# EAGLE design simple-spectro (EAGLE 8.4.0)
DELETE: MF
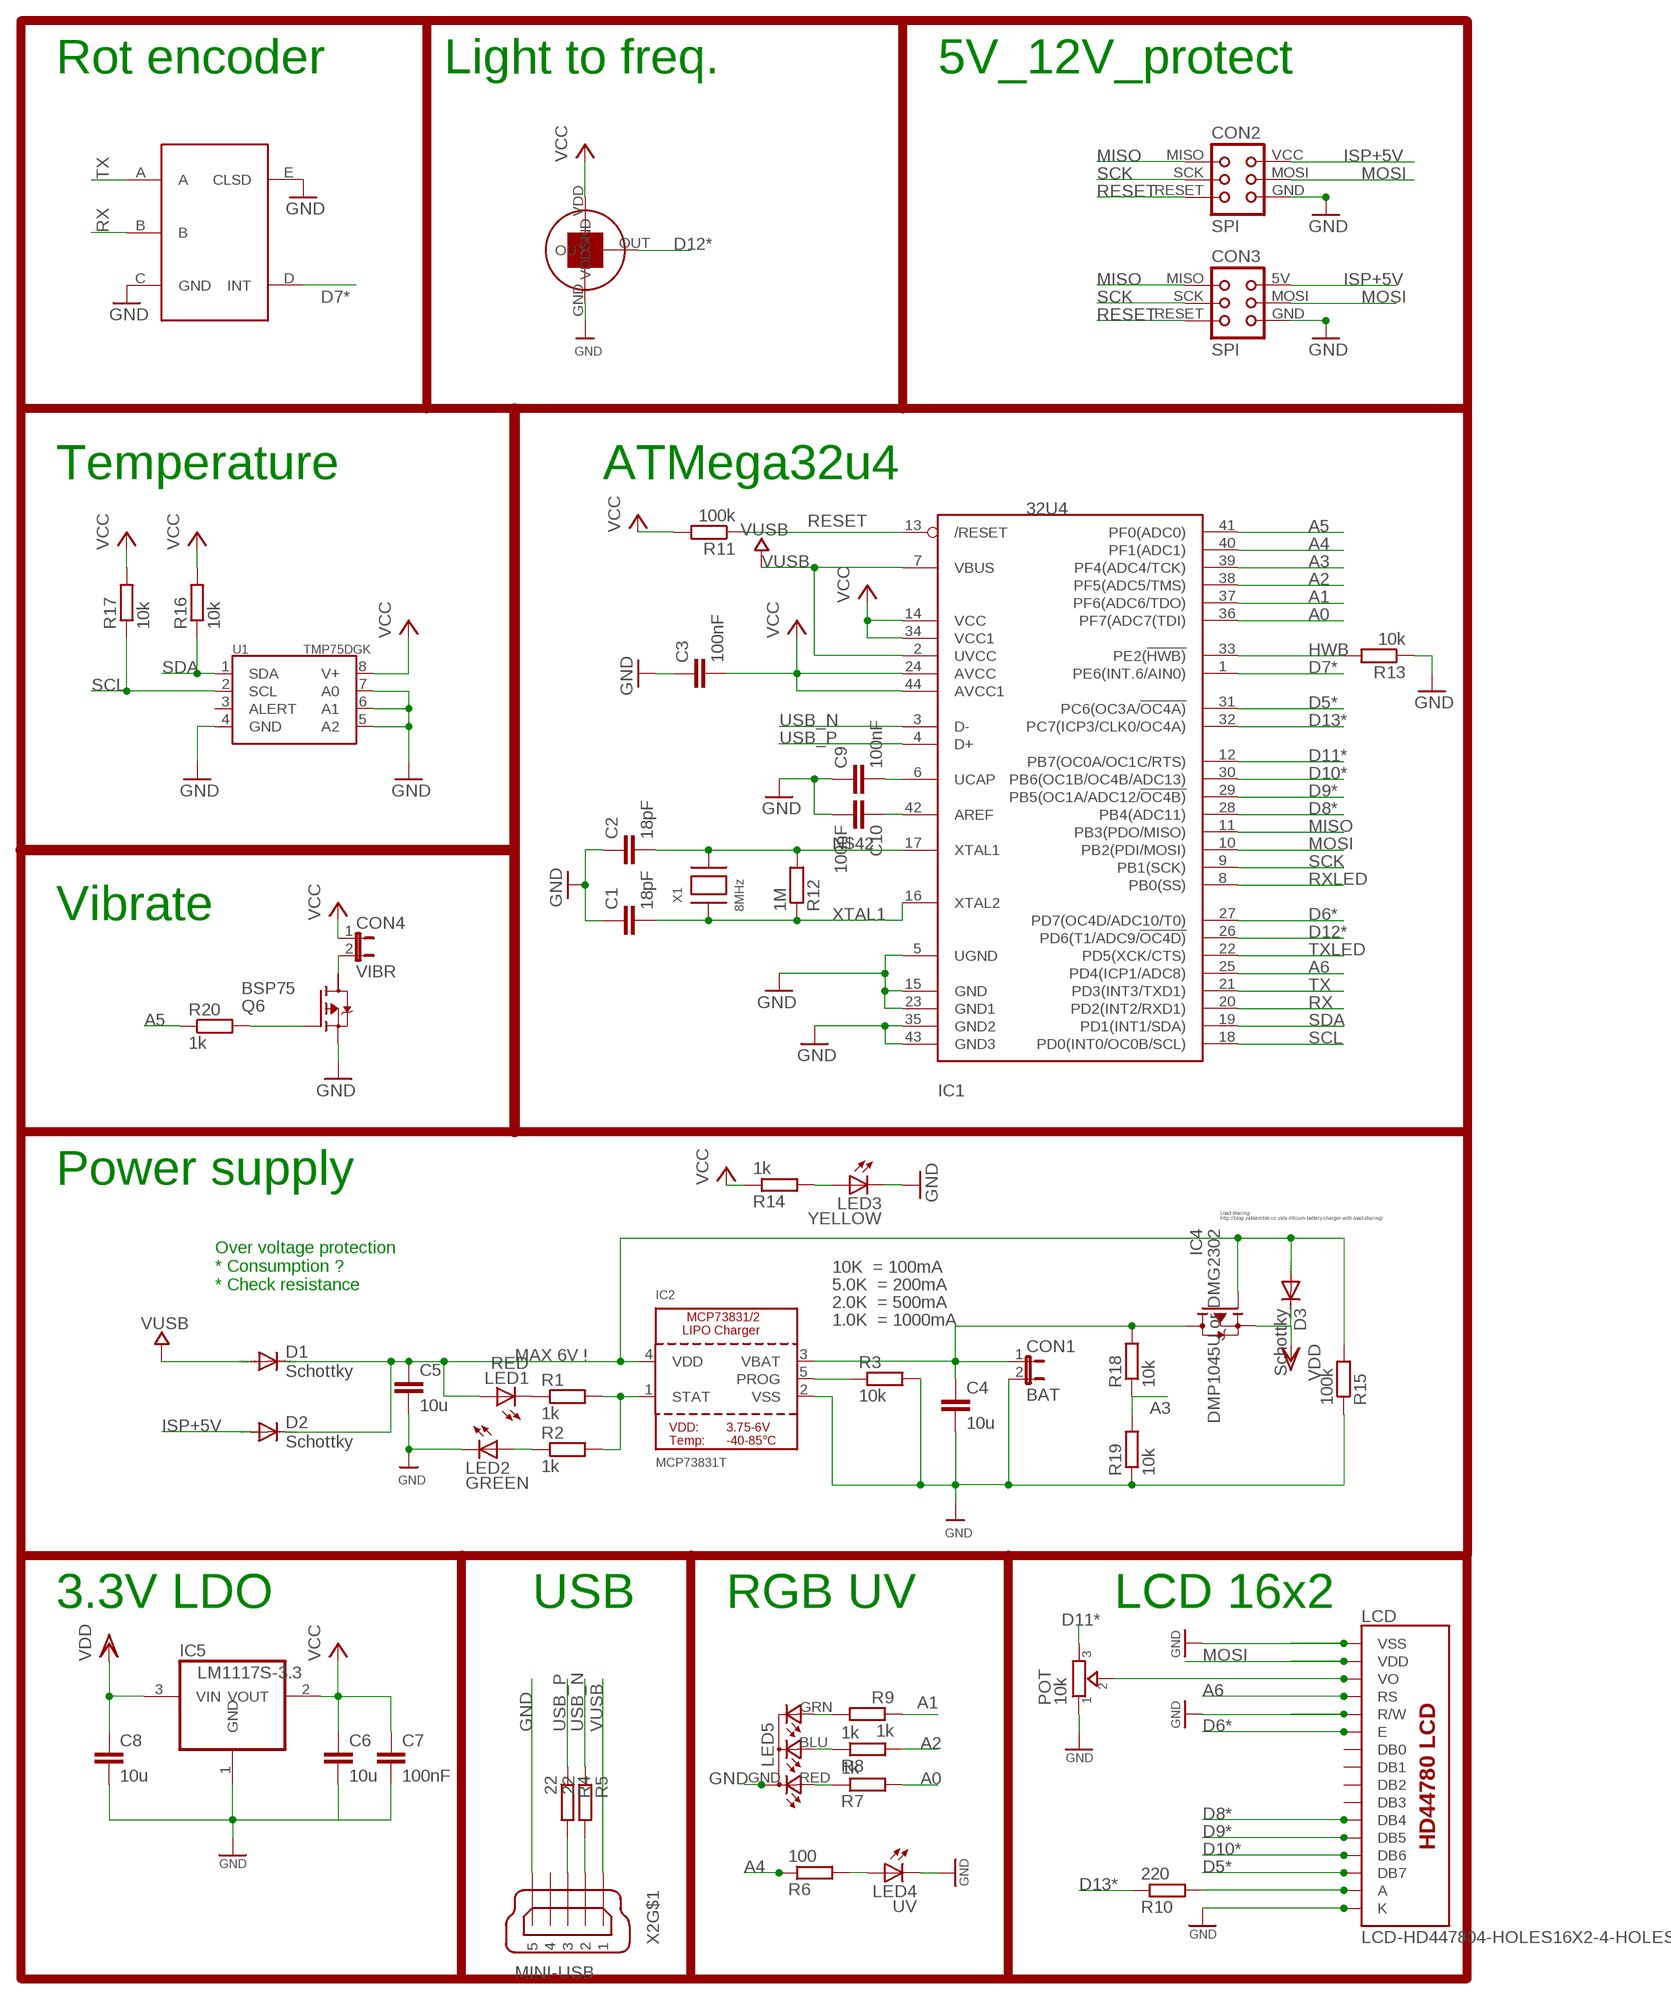
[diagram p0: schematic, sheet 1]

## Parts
C1  18pF  C-EUC0805K  [C0805K]
C2  18pF  C-EUC0805K  [C0805K]
C3  100nF  C-EUC0805K  [C0805K]
C4  10u  C-EUC0805K  [C0805K]
C5  10u  C-EUC0805K  [C0805K]
C6  10u  C-EUC0805K  [C0805K]
C7  100nF  C-EUC0805K  [C0805K]
C8  10u  C-EUC0805K  [C0805K]
C9  100nF  C-EUC0805K  [C0805K]
C10  100nF  C-EUC0805K  [C0805K]
CON1  BAT  JP1E  [JP1]
CON2  SPI  TINYISP  [TINYISP]
CON3  SPI  TINYISPT  [TC2030-MCP-NL]
CON4  VIBR  JP1E  [JP1]
D1  Schottky  MBR0520LT  [SOD123]
D2  Schottky  MBR0520LT  [SOD123]
D3  Schottky  MBR0520LT  [SOD123]
IC1  32U4  ATMEGA32U4-AU  [TQFP44]
IC2  MCP73831T  MCP73831/2  [SOT23-5]
IC4  DMP1045U or DMG2302  TRANSISTOR_FET_TSM2301CX  [SOT-23]
IC5  LM1117S-3.3  REG1117  [SOT223]
LCD  LCD-HD447804-HOLES16X2-4-HOLES  [LCD-16X2-4HOLES]
LED1  RED  LED1206  [LED-1206]
LED2  GREEN  LED1206  [LED-1206]
LED3  YELLOW  LED1206  [LED-1206]
LED4  UV  LED5MM  [LED5MM]
LED5  RGB-COMMON-CATHODE  [LED-TRICOLOR-THROUGHHOLE]
POT  10k  TRIMMER-3362P  [TRIMMER_3362P]
Q6  BSP75  BSP613P  [PG-SOT-223]
R1  1k  R-EU_R0805  [R0805]
R2  1k  R-EU_R0805  [R0805]
R3  10k  R-EU_R0805  [R0805]
R4  22  R-EU_R0805  [R0805]
R5  22  R-EU_R0805  [R0805]
R6  100  R-EU_R0805  [R0805]
R7  1k  R-EU_R0805  [R0805]
R8  1k  R-EU_R0805  [R0805]
R9  1k  R-EU_R0805  [R0805]
R10  220  R-EU_R0805  [R0805]
R11  100k  R-EU_R0805  [R0805]
R12  1M  R-EU_R0805  [R0805]
R13  10k  R-EU_R0805  [R0805]
R14  1k  R-EU_R0805  [R0805]
R15  100k  R-EU_R0805  [R0805]
R16  10k  R-EU_R0805  [R0805]
R17  10k  R-EU_R0805  [R0805]
R18  10k  R-EU_R0805  [R0805]
R19  10k  R-EU_R0805  [R0805]
R20  1k  R-EU_R0805  [R0805]
U1  TMP75DGK  [MSOP8]
U$1  EC11E  [EC11E]
U$7  TSL237  [TSL237]
X1  8MHz  XTALNX6035  [NX6035]
X2  MINI-USB  MINI-USB-SCHIELD-32005-201  [32005-201]

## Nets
A0: IC1.36(PF7(ADC7(TDI)) R7.2
A1: IC1.37(PF6(ADC6/TDO)) R9.1
A2: IC1.38(PF5(ADC5/TMS)) R8.2
A3: IC1.39(PF4(ADC4/TCK)) R18.1 R19.2
A4: IC1.40(PF1(ADC1)) R6.1
A5: IC1.41(PF0(ADC0)) R20.1
A6: IC1.25(PD4(ICP1/ADC8)) LCD.4(RS)
AREF: C10.1 IC1.42(AREF)
D5*: IC1.31(PC6(OC3A/!OC4A)) LCD.14(DB7)
D6*: IC1.27(PD7(OC4D/ADC10/T0)) LCD.6(E)
D7*: IC1.1(PE6(INT.6/AIN0)) U$1.D(INT)
D8*: IC1.28(PB4(ADC11)) LCD.11(DB4)
D9*: IC1.29(PB5(OC1A/ADC12/!OC4B)) LCD.12(DB5)
D10*: IC1.30(PB6(OC1B/OC4B/ADC13)) LCD.13(DB6)
D11*: IC1.12(PB7(OC0A/OC1C/RTS)) POT.3
D12*: IC1.26(PD6(T1/ADC9/!OC4D)) U$7.OUT
D13*: IC1.32(PC7(ICP3/CLK0/OC4A)) R10.1
GND [power]: C1.1 C2.1 C3.1 C4.2 C5.2 C6.2 C7.2 C8.2 C9.1 C10.2 CON1.2 CON2.GND CON3.GND IC1.5(UGND) IC1.15(GND) IC1.23(GND1) IC1.35(GND2) IC1.43(GND3) IC2.2(VSS) IC5.1(GND) LCD.1(VSS) LCD.5(R/W) LCD.16(K) LED2.C LED3.C LED4.K(C) LED5.GND(A2) POT.1 Q6.3(S) R3.2 R13.1 R15.1 R19.1 U1.4(GND) U1.5(A2) U1.6(A1) U1.7(A0) U$1.C(GND) U$1.E(CLSD) U$7.GND X2.5
HWB: IC1.33(PE2(!HWB)) R13.2
ISP+5V: CON2.VCC CON3.5V(VCC) D2.A
MISO: CON2.MISO CON3.MISO IC1.11(PB3(PDO/MISO))
MOSI: CON2.MOSI CON3.MOSI IC1.10(PB2(PDI/MOSI)) LCD.2(VDD)
N$1: C9.2 IC1.6(UCAP)
N$2: LCD.3(VO) POT.2
N$3: LED4.A R6.2
N$4: LED1.C R1.1
N$5: IC2.1(STAT) R1.2 R2.2
N$6: IC2.5(PROG) R3.1
N$7: LED2.A R2.1
N$8: Q6.1(G) R20.2
N$9: LED5.GRN(CGREEN) R9.2
N$10: LED5.BLU(CBLUE) R8.1
N$11: LCD.15(A) R10.2
N$12: LED3.A R14.2
N$13: LED5.RED(CRED) R7.1
N$14: CON4.2 Q6.2(D)
N$15: C5.1 D1.C D2.C D3.A IC2.4(VDD) IC4.1(G) LED1.A R15.2
N$42: C2.2 IC1.17(XTAL1) R12.2 X1.P$2
RESET: CON2.RESET CON3.RESET IC1.13(/RESET) R11.1
RX: IC1.20(PD2(INT2/RXD1)) U$1.B
RXLED: IC1.8(PB0(SS))
SCK: CON2.SCK CON3.SCK IC1.9(PB1(SCK))
SCL: IC1.18(PD0(INT0/OC0B/SCL)) R17.1 U1.2(SCL)
SDA: IC1.19(PD1(INT1/SDA)) R16.1 U1.1(SDA)
TX: IC1.21(PD3(INT3/TXD1)) U$1.A
TXLED: IC1.22(PD5(XCK/CTS))
USB_N: IC1.3(D-) R5.1
USB_P: IC1.4(D+) R4.1
USBC_N: R5.2 X2.2
USBC_P: R4.2 X2.3
VBAT1: C4.1 CON1.1 IC2.3(VBAT) IC4.3(D) R18.2
VCC: C3.2 C6.1 C7.1 CON4.1 IC1.14(VCC) IC1.24(AVCC) IC1.34(VCC1) IC1.44(AVCC1) IC5.2(VOUT) R11.2 R14.1 R16.2 R17.2 U1.8(V+) U$7.VDD
VDD [power]: C8.1 D3.C IC4.2(S) IC5.3(VIN)
VUSB: D1.A IC1.2(UVCC) IC1.7(VBUS) X2.1
XTAL1: C1.2 IC1.16(XTAL2) R12.1 X1.P$1
Unconnected: LCD.7(DB0) LCD.8(DB1) LCD.9(DB2) LCD.10(DB3) Q6.4(D) U1.3(ALERT) X2.4 X2.M1(S:S1) X2.M2(S:S2) X2.M3(S:S3) X2.M4(S:S4)

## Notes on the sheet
- Rot encoder | Light to freq. | 5V_12V_protect
- Temperature | ATMega32u4
- Vibrate
- Power supply
- Load sharing:
  http://blog.zakkemble.co.uk/a-lithium-battery-charger-with-load-sharing/
- 10K  = 100mA
- Over voltage protection
  * Consumption ?
  * Check resistance
- 5.0K  = 200mA
- 2.0K  = 500mA
- 1.0K  = 1000mA
- MAX 6V !
- 3.3V LDO | USB | RGB UV | LCD 16x2

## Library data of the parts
C1 C2 = rcl:C-EU: CAPACITOR, European symbol; ELECROW: C1797; LCSC: C1797; MPN: 77-VJ1206A180JXXPBC
C3 C9 C10 = rcl:C-EU: CAPACITOR, European symbol; ELECROW: C49678; LCSC: C49678; MPN: 80-C1206C104K5R
C4-C6 C8 = rcl:C-EU: CAPACITOR, European symbol; ELECROW: C15850; LCSC: C15850; MPN: 77-VJ1206V106ZXQTBC
C7 = rcl:C-EU: CAPACITOR, European symbol; ELECROW: C49678; LCSC: C77502; MPN: 80-C1206C104K5R
CON1 CON4 = jumper:JP1E: JUMPER
CON2 = lpatiny:TINYISP: CONNECTOR; OC_FARNELL: unknown; OC_NEWARK: unknown
CON3 = lpatiny:TINYISP: CONNECTOR
D1-D3 = diode:MBR0520LT: SCHOTTKY BARRIER RECTIFIER; LCSC: C82544; MPN: 621-1N5819HW-F
IC1 = adafruit:ATMEGA32U4: http://www.ladyada.net/library/eagle; LCSC: C44854; MPN: 556-ATMEGA32U4RC-AU
IC2 = microbuilder:MCP73831/2: MCP73831/2 LIPO Charger VDD: 3.75 - 6V Temp -40 - 85°C Programmable Charge Rate: 15-500mA NOTE: STAT is a tri-state logic output on the MCP73831 and an open-drain output on the MCP73832. SOT23-5 with 4.2V output and tri-state logic on STAT = MCP73831T-2ACI/OT; LCSC: C14879; MPN: 579-MCP73831T-3ACIOT
IC4 = dp_devices:TRANSISTOR_FET_TSM2301CX: 20V P-Channel Enhancement Mode MOSFET; LCSC: C96613; MPN: 621-DMP1045U-7
IC5 = burr-brown:REG1117: 800mA and 1A Low Dropout (LDO) Positive Regulator 1.8V, 2.5V, 2.85V, 3.3V, 5V, and Adj; LCSC: C126027; MPN: REG1117; OC_FARNELL: 1097566; OC_NEWARK: 14P6981
LCD = HD44780LCD:LCD-HD44780
LED1 = SparkFun:LED: LEDs; LCSC: C49018; MPN: 604-APT3216EC
LED2 = SparkFun:LED: LEDs; LCSC: C14641; MPN: 604-APTR3216SGC
LED3 = SparkFun:LED: LEDs; LCSC: C84273; MPN: 604-APTR3216YC
LED4 = SparkFun:LED: LEDs
LED5 = lpatiny:RGB-COMMON-CATHODE
POT = dp_devices:TRIMMER: Trimmer resistor
Q6 = infineon:BSP613P: SIPMOS (R) Small-Signal-Transistor P-Channel (2 Drain) Source: http://www.infineon.com/dgdl/BSP613P_Rev2.4.pdf; LCSC: C111029; OC_FARNELL: unknown; OC_NEWARK: unknown
R1 R2 R7-R9 R14 R20 = rcl:R-EU_: RESISTOR, European symbol; ELECROW: C17513; LCSC: C17513
R3 R13 R16-R19 = rcl:R-EU_: RESISTOR, European symbol; ELECROW: C17414; LCSC: C17414
R4 R5 = rcl:R-EU_: RESISTOR, European symbol; ELECROW: C17561; LCSC: C17561
R6 = rcl:R-EU_: RESISTOR, European symbol; ELECROW: C17408; LCSC: C17408; MPN: 667-ERJ-8GEYJ101V
R10 = rcl:R-EU_: RESISTOR, European symbol; ELECROW: C17557; LCSC: C17557
R11 R15 = rcl:R-EU_: RESISTOR, European symbol; ELECROW: C118844; LCSC: C118844; MPN: RC1206FR-07100KL
R12 = rcl:R-EU_: RESISTOR, European symbol; ELECROW: C17514; LCSC: C17514
U1 = ti_tmp:TMP75; LCSC: C94387
U$1 = lpatiny:EC11E: ALPS Rotary encoder
U$7 = lpatiny:TSL237
X1 = lpatiny:XTAL: Low cost SMT crystals, no capacitors included; LCSC: C122522; MPN: 729-F60800010
X2 = con-cypressindustries:MINI-USB-SCHIELD-: MINI USB-B Conector Source: www.cypressindustries.com; LCSC: C46391; MPN: 649-10033526-N3212LF

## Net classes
0 default: width 0.406 mm, clearance 0.25 mm
1 power: width 0.406 mm, drill 0.305 mm, clearance 0.25 mm
2 VIN: width 0.406 mm, clearance 0.25 mm
3 fine: width 0.406 mm, clearance 0.25 mm
4 aref: width 0.406 mm, clearance 0.25 mm

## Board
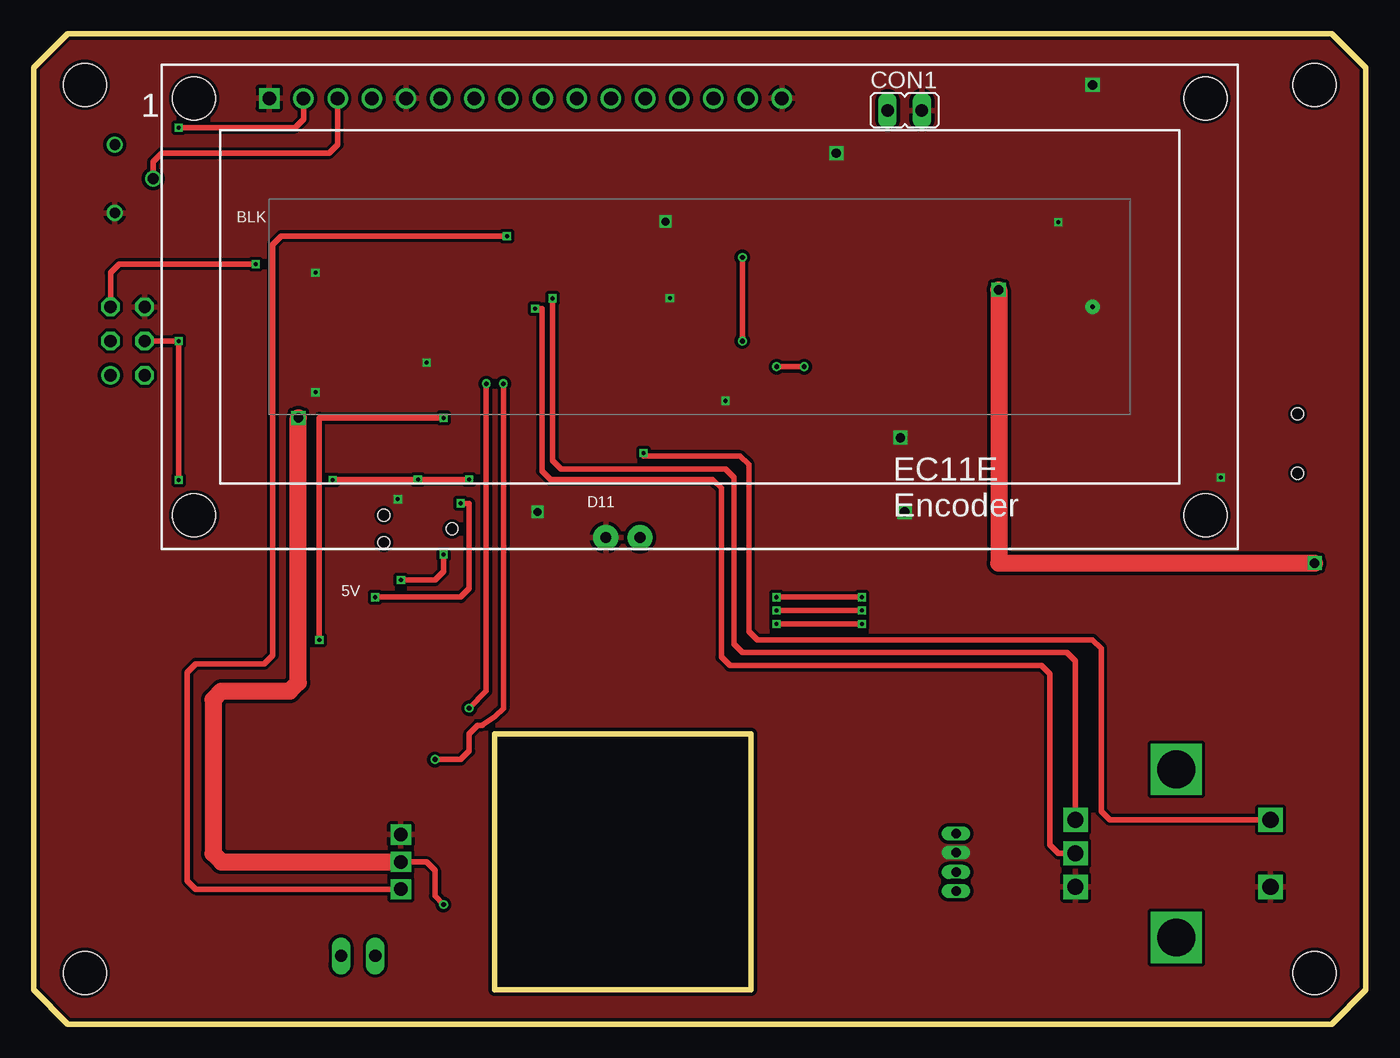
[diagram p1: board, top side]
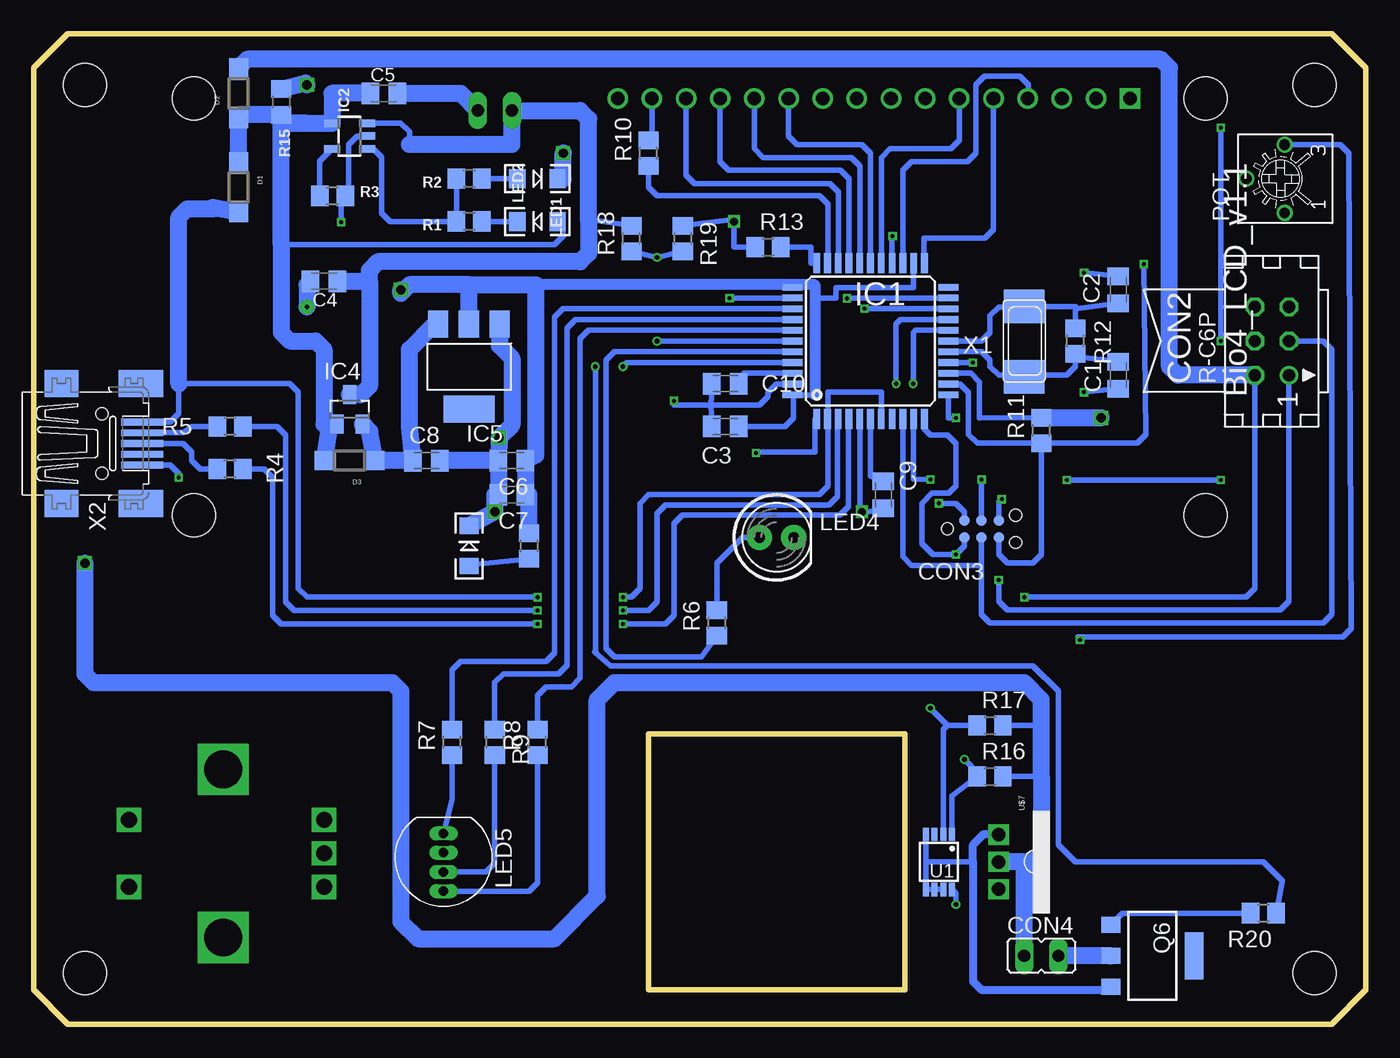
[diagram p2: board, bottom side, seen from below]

Size 99.06 x 73.66 mm. Coordinates in mm from the lower left corner, seen from the top.
Outline: 34.29,21.59 53.34,21.59 53.34,2.54 34.29,2.54 34.29,21.59
Outline: 0,71.12 0,2.54 2.54,0 96.52,0 99.06,2.54 99.06,71.12 96.52,73.66 2.54,73.66 0,71.12
Copper layers (1*2*15*16): Top 0.035mm / dielectric 0.2mm / layer 2 0.0175mm / dielectric 1.1mm / layer 15 0.0175mm / dielectric 0.2mm / Bottom 0.035mm
Design rules "SeeedStudio_DRU_no_angle_20130527": minimum track width 6mil, minimum drill 12mil, track to track 6mil, track to pad 6mil, pad to pad 6mil, via to via 6mil, smd to smd 0mil, copper to edge 10mil, drill to drill 10mil, minimum pad ring 6mil, minimum via ring 6mil, stop-mask expansion 2mil, vias tented up to drill 25mil, thermal gap 10mil
Holes 3.2 mm at 3.81,69.85 3.81,3.81 95.25,69.85 95.25,3.81

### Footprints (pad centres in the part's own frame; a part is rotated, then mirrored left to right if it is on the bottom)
C0805K = smd 1.3 x 1.6: 1 -1,0; 2 1,0
JP1 = drill 0.914 long: 1 0,-1.27; 2 0,1.27
TINYISP = drill 0.914 octagon: GND 2.54,1.27; MOSI 0,1.27; RESET 2.54,-1.27; SCK 0,-1.27; VCC -2.54,1.27 | drill 0.914: MISO -2.54,-1.27
TC2030-MCP-NL = smd 0.787 x 0.787: 5V 1.27,0.635; GND 3.81,0.635; MISO 1.27,-0.635; MOSI 2.54,0.635; RESET 3.81,-0.635; SCK 2.54,-0.635 | hole 0.889: 0,0; 5.08,-1.016; 5.08,1.016
SOD123 = smd 1.4 x 1.4: A 1.9,0; C -1.9,0
TQFP44 = smd 1.5 x 0.5: 1 -5.8,4; 2 -5.8,3.2; 3 -5.8,2.4; 4 -5.8,1.6; 5 -5.8,0.8; 6 -5.8,0; 7 -5.8,-0.8; 8 -5.8,-1.6; 9 -5.8,-2.4; 10 -5.8,-3.2; 11 -5.8,-4; 23 5.8,-4; 24 5.8,-3.2; 25 5.8,-2.4; 26 5.8,-1.6; 27 5.8,-0.8; 28 5.8,0; 29 5.8,0.8; 30 5.8,1.6; 31 5.8,2.4; 32 5.8,3.2; 33 5.8,4 | smd 0.5 x 1.5: 12 -4,-5.8; 13 -3.2,-5.8; 14 -2.4,-5.8; 15 -1.6,-5.8; 16 -0.8,-5.8; 17 0,-5.8; 18 0.8,-5.8; 19 1.6,-5.8; 20 2.4,-5.8; 21 3.2,-5.8; 22 4,-5.8; 34 4,5.8; 35 3.2,5.8; 36 2.4,5.8; 37 1.6,5.8; 38 0.8,5.8; 39 0,5.8; 40 -0.8,5.8; 41 -1.6,5.8; 42 -2.4,5.8; 43 -3.2,5.8; 44 -4,5.8
SOT23-5 = smd 0.55 x 1.2: 1 -0.95,-1.3; 2 0,-1.3; 3 0.95,-1.3; 4 0.95,1.3; 5 -0.95,1.3
SOT-23 = smd 1 x 1.4: 1 -0.95,-1.1; 2 0.95,-1.1; 3 0,1.1
SOT223 = smd 1.499 x 2.007: 1 -2.261,-3.15; 2 0.025,-3.15; 3 2.311,-3.15 | smd 3.81 x 2.007: 4 0,3.15
LCD-16X2-4HOLES = drill 1.016 square: 1 -32,15.5 | drill 1.016: 2 -29.46,15.5; 3 -26.92,15.5; 4 -24.38,15.5; 5 -21.84,15.5; 6 -19.3,15.5; 7 -16.76,15.5; 8 -14.22,15.5; 9 -11.68,15.5; 10 -9.14,15.5; 11 -6.6,15.5; 12 -4.06,15.5; 13 -1.52,15.5; 14 1.02,15.5; 15 3.56,15.5; 16 6.1,15.5 | hole 3.2: -37.6,15.5; -37.6,-15.5; 37.6,-15.5; 37.6,15.5
LED-1206 = smd 1.2 x 1.4: A -1.5,0; C 1.5,0
LED5MM = drill 0.813 pad 1.88: A -1.27,0; K 1.27,0
LED-TRICOLOR-THROUGHHOLE = drill 0.7 long: BLU 2.175,0; GND -0.682,0; GRN 0.746,0; RED -2.111,0
TRIMMER_3362P = drill 0.8: 1 -2.54,-0.31; 2 0,2.54; 3 2.54,-0.31
PG-SOT-223 = smd 1.2 x 1.4: 1 -2.311,-3.099; 2 0,-3.099; 3 2.311,-3.099 | smd 3.5 x 1.4: 4 0,3.099
R0805 = smd 1.3 x 1.5: 1 -0.95,0; 2 0.95,0
MSOP8 = smd 0.45 x 1: 1 -0.975,-2.05; 2 -0.325,-2.05; 3 0.325,-2.05; 4 0.975,-2.05; 5 0.975,2.05; 6 0.325,2.05; 7 -0.325,2.05; 8 -0.975,2.05
EC11E = drill 1.2 square: A -2.5,0; B 0,0; C 2.5,0; D -2.5,14.5; E 2.5,14.5 | drill 2.8 square: P$1 6.25,7.5; P$2 -6.25,7.5
TSL237 = drill 1 pad 1.27 square: GND -2.032,-2.54; OUT 2.032,-2.54; VDD 0,-2.54
NX6035 = smd 2.5 x 3: P$1 2.665,0; P$2 -2.565,0
32005-201 = smd 3.1 x 0.5: 1 3,1.6; 2 3,0.8; 3 3,0; 4 3,-0.8; 5 3,-1.6 | smd 2.5 x 2: M1 -3,-4.45; M2 -3,4.45 | smd 3.3 x 2: M3 2.9,4.45; M4 2.9,-4.45 | hole 0.9: 0,2.2; 0,-2.2

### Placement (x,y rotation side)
C1  18.41,48.26 90 bottom
C2  18.41,54.61 270 bottom
C3  47.62,44.45 0 bottom
C4  77.47,55.24 180 bottom
C5  73.03,69.22 0 bottom
C6  63.5,41.91 180 bottom
C7  63.5,39.37 180 bottom
C8  69.85,41.91 0 bottom
C9  35.88,39.37 90 bottom
C10  47.62,47.62 180 bottom
CON1  64.77,67.94 270 top
CON2  6.99,50.8 90 bottom
CON3  31.11,36.83 0 bottom
CON4  24.13,5.08 270 bottom
D1  83.82,62.23 270 bottom
D2  83.82,69.22 90 bottom
D3  75.56,41.91 180 bottom
IC1  36.83,50.8 90 bottom
IC2  75.56,66.04 90 bottom
IC4  75.56,45.72 0 bottom
IC5  66.67,48.9 180 bottom
LCD  49.53,53.34 0 top
LED1  61.59,59.69 180 bottom
LED2  61.59,62.87 0 bottom
LED3  66.67,35.56 90 bottom
LED4  43.81,36.2 0 bottom
LED5  68.58,12.06 270 bottom
POT  6.35,62.87 90 bottom
Q6  15.88,5.08 270 bottom
R1  66.67,59.69 180 bottom
R2  66.67,62.87 180 bottom
R3  76.83,61.59 0 bottom
R4  84.45,41.27 180 bottom
R5  84.45,44.45 180 bottom
R6  48.26,29.84 90 bottom
R7  67.94,20.95 90 bottom
R8  61.59,20.95 90 bottom
R9  64.77,20.95 270 bottom
R10  53.34,64.77 90 bottom
R11  24.13,44.16 90 bottom
R12  21.59,50.8 90 bottom
R13  44.45,57.78 0 bottom
R14  62.23,35.56 270 bottom
R15  80.64,68.58 270 bottom
R16  27.94,18.41 0 bottom
R17  27.94,22.23 0 bottom
R18  54.61,58.42 90 bottom
R19  50.8,58.42 270 bottom
R20  7.62,8.26 180 bottom
U1  31.75,12.06 180 bottom
U$1  77.47,12.7 270 top
U$7  24.77,12.06 270 bottom
X1  25.4,50.8 270 bottom
X2  93.98,43.18 0 bottom

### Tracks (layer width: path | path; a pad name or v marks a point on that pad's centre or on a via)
A0
  Bottom 0.406: IC1.36 59.69,53.2 60.33,52.56 60.33,27.61 60.96,26.98 67.31,26.98 67.94,26.34 R7.2
A1
  Bottom 0.406: IC1.37 58.78,52.4 59.41,51.77 59.41,26.67 60.05,26.04 64.14,26.04 64.77,25.4 R9.1
A2
  Bottom 0.406: IC1.38 57.78,51.6 58.42,50.97 58.42,25.73 59.05,25.09 60.96,25.09 61.59,24.46 R8.2
A3  (via drill 0.35)
  Top 0.406: v52.7,50.8 v52.7,57.02
  Bottom 0.406: R19.2 v52.7,57.02 R18.1 | IC1.39 v52.7,50.8
A4
  Bottom 0.406: 42.63,50.04 IC1.40 55.88,50 56.52,49.37 56.52,27.94 55.88,27.3 49.4,27.3 R6.1
A5  (via drill 0.35)
  Top 0.406: v55.24,48.9 v57.3,48.9
  Bottom 0.406: R20.1 6.22,10.66 7.62,12.06 21.59,12.06 22.86,13.34 22.86,24.77 24.74,26.65 56.15,26.65 57.05,27.42 | 57.05,27.42 57.34,27.67 | IC1.41 54.93,49.21 v55.24,48.9 | 57.05,27.42 57.3,27.66 v57.3,48.9
A6
  Bottom 0.406: LCD.4 25.08,68.84 25.08,69.85 25.72,70.48 28.36,70.48 29,69.85 29,64.77 29.64,64.14 33.8,64.14 34.43,63.5 IC1.25
AREF
  Bottom 0.406: IC1.42 46.23,48.4 C10.1
D5*
  Bottom 0.406: 39.24,56.6 IC1.31 39.23,61.87 39.87,62.5 49.91,62.5 50.55,63.14 LCD.14
D6*
  Bottom 0.406: IC1.27 36.03,64.45 35.4,65.09 30.86,65.09 30.23,65.72 LCD.6
D7*  (via drill 0.3)
  Top 0.406: U$1.D 80.01,15.2 79.38,15.84 79.38,27.94 78.74,28.57 53.81,28.57 53.17,29.21 53.17,41.6 52.54,42.24 45.34,42.24 v45.34,42.48
  Bottom 0.406: IC1.1 40.96,45 40.96,42.55 45.34,42.55 v45.34,42.48 | 91.97,14.93 U$1.D
D8*
  Bottom 0.406: LCD.11 42.93,66.04 42.3,65.41 37.47,65.41 36.83,64.77 IC1.28
D9*
  Bottom 0.406: LCD.12 45.47,65.09 44.84,64.45 38.27,64.45 37.63,63.82 IC1.29
D10*
  Bottom 0.406: LCD.13 48.01,64.14 47.38,63.5 39.06,63.5 38.43,62.87 IC1.30
D11*  (via drill 0.3)
  Top 0.406: v21.25,28.57 21.25,45.09 v30.48,45.09
  Bottom 0.406: POT.3 1.9,65.41 1.27,64.77 1.1,29.43 1.74,28.8 21.42,28.8 v21.25,28.57 | v30.48,45.09 31.03,45.09 IC1.12
D12*  (via drill 0.3)
  Top 0.406: v35.19,58.61 18.41,58.61 17.78,57.98 17.78,27.43 17.14,26.8 12.06,26.8 11.43,26.16 11.43,10.67 12.06,10.03 U$7.OUT
  Bottom 0.406: IC1.26 35.24,58.51 35.19,58.51 v35.19,58.61
D13*
  Bottom 0.406: IC1.32 40.01,56.6 40.01,60.96 40.64,61.59 52.7,61.59 53.34,62.23 R10.1
GND  (via drill 0.3, 0.35 pad 1.05, 0.6, 0.7)
  Bottom 0.406: 49.02,47.6 C10.2 48.68,46.04 | 48.68,46.04 C3.1 | IC1.43 43.81,47.6 44.45,46.97 44.45,46.67 45.09,46.04 48.68,46.04 | v51.44,46.35 51.44,46.04 48.68,46.04 | C9.1 37.47,37.97 | IC1.5 37.63,37.97 37.47,37.97 | LCD.5 27.69,59.08 28.32,58.45 32.85,58.45 32.85,56.6 IC1.23 | 64.77,41.91 C6.2 | C7.2 64.77,39.37 | X2.5 88.9,41.58 88.27,40.95 v88.27,40.64 | IC1.35 v47.3,54 | C2.1 v20.95,55.88 | IC1.15 v29.22,49.2 | v29.22,49.2 | CON3.GND 27.3,38.81 v27.08,39.04 | R13.1 46.99,57.78 v46.99,59.69 47.12,59.82 R19.1 | 37.47,37.97 v37.47,38.1 | C1.1 v20.95,46.99 | v76.2,59.64 76.2,61.59 R3.2 75.65,61.59 75.65,65.41 75.01,66.04 IC2.2 | U1.7 U1.6 U1.5 32.73,12.06 | 32.73,12.06 32.73,13.4 32.75,13.43 32.75,14.09 U1.4 | 32.73,12.06 29.21,12.06
  Bottom 0.61: U$7.GND 28.45,14.1 29.21,13.34 29.21,12.06 29.21,3.17 28.57,2.54 19.2,2.54 Q6.3
  Bottom 1.27: LED2.C 59.69,62.87 v59.69,64.77 | C6.2 v64.45,43.62 63.5,44.57 63.5,49.53 64.41,50.44 IC5.1 | C6.2 C8.2 | C6.2 C7.2 | LED3.C v64.77,38.1 64.77,39.37 | R15.1 78.87,69.98 v78.74,69.85 | C5.2 67.31,69.22 CON1.2 | C4.2 78.74,54.98 v78.74,53.34
  pour Top: 0,71.12 0,2.54 2.54,0 96.52,0 99.06,2.54 99.06,71.12 96.52,73.66 2.54,73.66
HWB
  Bottom 0.406: IC1.33 41.27,56.6 41.27,57.78 R13.2
ISP+5V  (via drill 0.3)
  Top 0.406: v31.75,38.73 32.38,38.73 32.38,32.38 31.75,31.75 v25.4,31.75
  Bottom 0.406: CON3.5V 29.84,38.1 30.48,38.73 v31.75,38.73 | v25.4,31.75 8.89,31.75 8.26,32.38 CON2.VCC
  Bottom 1.27: CON2.VCC 13.97,48.26 14.61,48.9 14.61,71.12 15.24,71.75 83.19,71.75 D2.A
MISO  (via drill 0.3)
  Top 0.406: v27.3,33.02 29.84,33.02 30.48,33.66 v30.48,34.92
  Bottom 0.406: CON3.MISO 29.84,35.56 v30.48,34.92 32.2,34.92 33.02,35.75 33.02,38.73 32.26,39.49 30.99,39.49 30.48,40.01 30.48,43.18 31.11,43.81 32.38,43.81 32.83,44.26 IC1.11 | CON2.MISO 5.71,31.42 6.35,30.79 26.67,30.79 27.3,31.42 v27.3,33.02
MOSI  (via drill 0.3)
  Top 0.406: v32.38,40.5 v28.57,40.5 22.23,40.5 v22.23,40.47 | CON2.MOSI v10.79,50.8 v10.79,40.47 | v10.79,66.67 19.43,66.67 20.07,67.31 LCD.2
  Bottom 0.406: CON3.MOSI v28.57,40.5 | v10.79,50.8 v10.79,66.67 | v22.23,40.47 v10.79,40.47 | IC1.10 33.63,40.52 v32.38,40.5
N$1
  Bottom 0.406: C9.2 36.83,40.77 IC1.6
N$2
  Top 0.406: POT.2 8.89,64.14 9.53,64.77 21.98,64.77 22.61,65.41 LCD.3
  Bottom 0.406: LCD.3
N$3
  Bottom 0.406: R6.2 48.26,34.29 46.35,36.2 LED4.A
N$4
  Bottom 0.406: LED1.C R1.1
N$5
  Bottom 0.406: R2.2 R1.2 72.56,59.69 73.19,60.33 73.19,64.45 73.83,65.09 IC2.1
N$6
  Bottom 0.406: IC2.5 77.78,64.17 R3.1
N$7
  Bottom 0.406: R2.1 LED2.A
N$8
  Bottom 0.406: Q6.1 18.11,8.26 R20.2
N$9
  Bottom 0.406: LED5.GRN 65.41,11.32 64.77,11.95 R9.2
N$10
  Bottom 0.406: LED5.BLU 62.23,9.89 61.59,10.53 R8.1
N$11
  Bottom 0.406: LCD.15 53.09,66.42 R10.2
N$12
  Bottom 0.406: R14.2 66.67,34.16 LED3.A
N$13
  Bottom 0.406: R7.1 67.94,16.72 LED5.RED
N$14
  Bottom 1.27: Q6.2 CON4.2
N$15
  Bottom 0.406: 77.06,44.62 IC4.1 | LED1.A 59.69,59.69 59.69,58.59 60.33,57.96 80.64,57.96
  Bottom 1.27: D1.C D2.C 83.82,67.63 R15.2 80.64,66.99 78.76,66.99 | 77.06,44.62 D3.A | 77.06,44.62 77.47,44.62 77.47,50.16 78.11,50.8 80.01,50.8 80.64,51.44 80.64,57.96 80.64,66.97 78.76,66.99 | 78.76,66.99 IC2.4 76.86,69.22 C5.1
N$42
  Bottom 0.406: IC1.17 28.57,50.8 27.94,51.44 27.94,52.7 27.3,53.34 25.4,53.34 X1.P$2 21.59,53.37 | 21.59,53.37 R12.2 | C2.2 21.43,53.21 21.59,53.37
RESET  (via drill 0.3)
  Top 0.406: v16.51,56.52 6.35,56.52 5.71,55.88 CON2.RESET
  Bottom 0.406: IC1.13 30.18,47.6 29.54,46.97 29.54,43.84 28.9,43.21 R11.1 | CON3.RESET 27.3,34.92 26.67,34.29 24.77,34.29 24.13,34.92 R11.1 | R11.1 16.98,43.21 16.35,43.85 v16.51,56.52
RX  (via drill 0.3)
  Top 0.406: v37.27,53.21 37.8,53.21 37.8,41.13 38.43,40.5 50.49,40.5 51.13,39.87 51.13,27.3 51.77,26.67 74.93,26.67 75.56,26.04 75.56,13.34 76.2,12.7 U$1.B
  Bottom 0.406: IC1.20 34.1,53.2 v37.27,53.21
SCK
  Bottom 0.406: CON3.SCK 28.57,34.12 | 28.57,34.12 33.8,34.12 34.43,34.76 IC1.9 | CON2.SCK 3.17,50.8 2.54,50.16 2.54,30.48 3.17,29.84 27.94,29.84 28.57,30.48 28.57,34.12
SCL  (via drill 0.35)
  Top 0.406: v33.66,47.62 33.66,42.55 33.66,24.77 v32.38,23.5
  Bottom 0.406: U1.2 31.43,21.91 31.11,22.23 | 31.11,22.23 R17.1 | IC1.18 33.49,51.6 33.66,51.44 v33.66,47.62 | 31.11,22.23 v32.38,23.5
SDA  (via drill 0.35)
  Top 0.406: v34.92,47.62 34.92,23.5 34.31,22.89 33.38,22.25 33.36,22.23 33.02,22.23 32.38,21.59 32.38,20.32 31.75,19.68 v29.84,19.68
  Bottom 0.406: U1.1 30.77,16.98 R16.1 29.34,19.18 v29.84,19.68 | IC1.19 34.59,52.4 34.92,52.07 v34.92,47.62
TX  (via drill 0.3)
  Top 0.406: v38.59,53.98 38.59,41.91 39.23,41.27 51.44,41.27 52.07,40.64 52.07,28.27 52.7,27.64 76.83,27.64 77.47,27 U$1.A
  Bottom 0.406: IC1.21 v38.59,53.98
USB_N  (via drill 0.3)
  Top 0.406: v55.24,30.76 v61.58,30.76
  Bottom 0.406: IC1.3 39.29,45 39.29,39.25 39.93,38.61 52.07,38.61 52.7,37.98 52.7,31.39 53.34,30.76 v55.24,30.76 | v61.58,30.76 79.69,30.76 80.33,31.39 80.33,43.81 80.96,44.45 R5.1
USB_P  (via drill 0.3)
  Top 0.406: v55.24,29.77 v61.58,29.77
  Bottom 0.406: v61.58,29.77 80.64,29.77 81.28,30.4 81.28,40.64 81.92,41.27 R4.1 | IC1.4 38.47,45 38.47,38.49 39.1,37.86 50.8,37.86 51.44,37.22 51.44,30.4 52.07,29.77 v55.24,29.77
USBC_N
  Bottom 0.406: X2.2 87.94,43.98 87.3,44.45 R5.2
USBC_P
  Bottom 0.406: X2.3 87.94,43.18 87.3,42.55 87.3,41.91 86.67,41.27 R4.2
VBAT1
  Bottom 0.406: IC2.3 71.75,66.99 71.12,66.36 71.12,65.41 | R18.2 57.66,59.82 57.78,59.69
  Bottom 1.27: 71.12,65.41 63.5,65.41 CON1.1 58.42,67.94 57.78,67.31 57.78,59.69 57.78,57.32 58.42,56.69 73.45,56.69 74.08,56.05 74.08,55.24 | 74.08,55.24 74.08,47.44 74.72,46.81 75.56,46.81 IC4.3 | C4.1 74.08,55.24
VCC  (via drill 0.35, 0.7)
  Top 0.406: U$7.VDD 29.21,12.06 29.84,11.43 29.84,9.53 v30.48,8.89
  Top 1.27: v71.75,54.61 71.75,34.29 v95.25,34.29 | v19.68,45.09 19.68,25.4 19.05,24.77 13.97,24.77 13.34,24.13 13.34,12.7 13.97,12.06 U$7.VDD
  Bottom 0.406: C3.2 43.18,44.45 42.55,45.09 42.55,46.8 IC1.44 40.98,46.8 40.8,53.98 | IC1.14 29.38,48.4 28.74,47.77 28.74,45.06 R11.2 | 40.8,53.98 40.8,54.8 IC1.34 | IC1.24 33.66,56.6 33.66,54.77 39.4,54.77 39.4,53.98 40.8,53.98 | R17.2 24.13,22.23 | R16.2 24.13,18.41 | v30.48,8.89 30.48,9.72 U1.8
  Bottom 0.813: 61.72,54.98 40.98,54.98 40.98,46.8
  Bottom 1.27: R14.1 62.23,39.37 C7.1 C6.1 61.72,42.29 61.72,54.98 66.67,54.98 | 66.67,54.98 71.12,54.98 71.75,54.34 v71.75,54.61 | v95.25,34.29 95.25,26.04 94.61,25.4 72.39,25.4 71.75,24.77 71.75,7.62 70.48,6.35 60.33,6.35 57.15,9.53 57.15,24.13 55.88,25.4 25.4,25.4 24.13,24.13 24.13,22.23 24.13,18.41 24.13,12.7 24.77,12.06 25.4,12.06 | v19.68,45.09 24.13,45.09 R11.2 | 25.4,12.06 U$7.VDD | CON4.1 25.4,12.06 | IC5.2 66.67,52.07 66.67,54.98
VDD
  Bottom 1.27: IC4.2 74.06,44.07 D3.C C8.1 71.12,44.45 71.12,50.16 69.24,52.05 IC5.3
VUSB  (via drill 0.3)
  Top 0.406: v55.24,31.75 v61.58,31.75
  Bottom 0.406: 40.01,45 40.01,46.99 36.03,46.99 IC1.7 | IC1.2 40.01,45 | 40.01,45 40.01,40.01 40.64,39.37 53.34,39.37 53.98,38.73 53.98,32.38 54.61,31.75 v55.24,31.75 | v61.58,31.75 78.74,31.75 79.38,32.38 79.38,46.99 80.01,47.62 88.27,47.62 88.27,45.41 88.9,44.78 X2.1 | 85.72,60.73 85.72,60.63
  Bottom 1.27: 88.27,47.62 88.27,59.99 87.63,60.63 85.72,60.63 | D1.A 85.72,60.73
XTAL1
  Bottom 0.406: 25.4,48.26 22.23,48.26 21.59,48.9 R12.1 21.59,49.66 C1.2 | 25.4,48.26 X1.P$1 | 25.4,48.26 27.3,48.26 27.94,48.9 27.94,49.37 28.57,50 IC1.16

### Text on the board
tNames: 1 | BLK | D11 | EC11E / Encoder | 5V
bNames: Bio4_LCD_v1.1
tValues: Simple spectro / V 1.4.0
bValues: Simple spectro / V1.4.0

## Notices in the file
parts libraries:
lpatiny: ©2009 ROFA.cz - modified and updated by Robert Darlington ‹rdarlington@gmail.com›
microbuilder: This work is placed in the public domain, and may be freely used for commercial and non-commercial work with the following conditions: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
